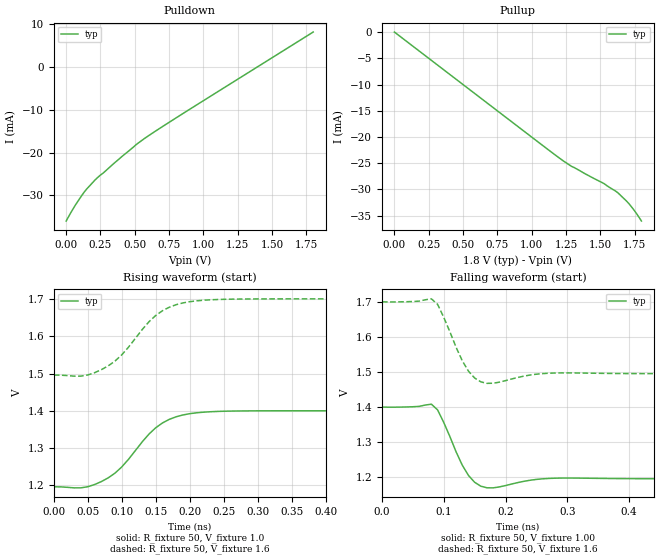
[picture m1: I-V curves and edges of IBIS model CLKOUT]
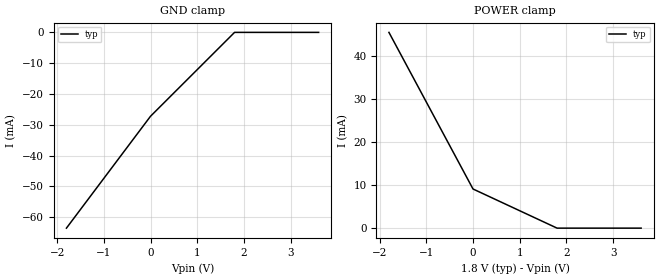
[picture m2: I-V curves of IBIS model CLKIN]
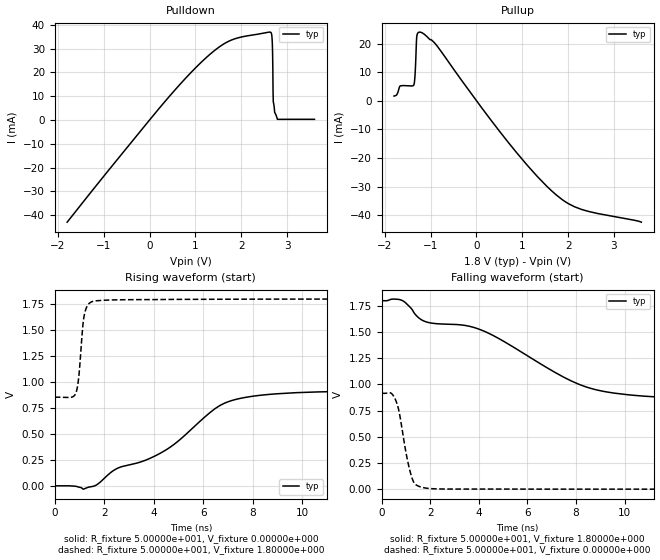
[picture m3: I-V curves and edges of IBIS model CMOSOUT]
|This Model applies to CDCL1810 and CDCL1810A Clock Buffers
[IBIS Ver] 4.0
[Comment char] |_char
[File Name] cdcl1810a.ibs
[File Rev] 2.0
[Source] Texas Instruments, Inc. Created from TISpice model
[Date] March 01, 2006
[Disclaimer]
|*   Property of Texas Instruments Incorporated.  Unauthorized  *
|*   reproduction and/or distribution is strictly prohibited.   *
|*   This product is protected under copyright law.   *
|*   (C) Copyright 2006, Texas Instruments Inc.,   *
|*   All Rights Reserved   *
|*   UNLESS THERE IS A SIGNED, WRITTEN AGREEMENT TO THE   *
|*   CONTRARY, TEXAS INSTRUMENTS ("TI") IS PROVIDING THE SPICE  *
|*   MODELS "AS IS" AND WITHOUT ANY WARRANTY, EXPRESSED OR   *
|*   IMPLIED.  TI assumes no liability for:   *
|*   1) the accuracy of the IBIS models provided to your   *
|*   company;   *
|*   2) the proper functioning of these IBIS models in your   *
|*   design or for any resulting applications; or   *
|*   3) infringement of patents, copyrights or intellectual   *
|*   property rights resulting from your use of these   *
|*   IBIS models.   *
|*   TI provides IBIS Models as a service to our customers.   *
|*   You and your company shall not distribute, sell or give   *
|*   these models to anyone else without prior written   *
|*   permission from TI.   *
|*   TI reserves the right to make changes to our products or   *
|*   to discontinue any semiconductor product or service   *
|*   without notice, and advises our customers to obtain the   *
|*   latest version of relevant information to verify, before   *
|*   placing orders, that the information being relied on is   *
|*   current.   *
|*   Please be aware that your receipt and use of the IBIS   *
|*   information provided shall serve as acceptance of these   *
|*   terms and conditions.  If you do not accept these terms,   *
|*   you should return or destroy the IBIS models and any   *
|*   other accompanying information immediately.   *
[Component] CDCL1810A
[Manufacturer] Texas Instruments, Inc.
[Package]
| variable   typ   min  max
R_pkg   0.175ohm   NA   NA
L_pkg   2.081nH   NA   NA
C_pkg   0.045pF   NA   NA
[Pin]   signal_name   model_name   R_pin   L_pin   C_pin
2   AVDD   POWER   NA   NA   NA
3   CLKP   CLKIN   NA   NA   NA
4   CLKN   CLKIN   NA   NA   NA
5   AVDD   POWER   NA   NA   NA
6   YP0   CLKOUT   NA   NA   NA
7   YN0   CLKOUT   NA   NA   NA
8   VDD   POWER   NA   NA   NA
9   YP1   CLKOUT   NA   NA   NA
10   YN1   CLKOUT   NA   NA   NA
11   VDD   POWER   NA   NA   NA
12   GND   GND   NA   NA   NA
13   STATUS   CMOSOUT   NA   NA   NA
14   VDD   POWER   NA   NA   NA
15   YP2   CLKOUT   NA   NA   NA
16   YN2   CLKOUT   NA   NA   NA
17   VDD   POWER   NA   NA   NA
18   YP3   CLKOUT   NA   NA   NA
19   YN3   CLKOUT   NA   NA   NA
20   VDD   POWER   NA   NA   NA
21   YP4   CLKOUT   NA   NA   NA
22   YN4   CLKOUT   NA   NA   NA
23   VDD   POWER   NA   NA   NA
24   SCL   CMOSIN   NA   NA   NA
25   SDA   CMOSIO   NA   NA   NA
26   VDD   POWER   NA   NA   NA
27   YP5   CLKOUT   NA   NA   NA
28   YN5   CLKOUT   NA   NA   NA
29   VDD   POWER   NA   NA   NA
30   YP6   CLKOUT   NA   NA   NA
31   YN6   CLKOUT   NA   NA   NA
32   VDD   POWER   NA   NA   NA
33   YP7   CLKOUT   NA   NA   NA
34   YN7   CLKOUT   NA   NA   NA
35   VDD   POWER   NA   NA   NA
36   ADD0   CMOSIN   NA   NA   NA
37   ADD1   CMOSIN   NA   NA   NA
38   VDD   POWER   NA   NA   NA
39   YN8   CLKOUT   NA   NA   NA
40   YP8   CLKOUT   NA   NA   NA
41   VDD   POWER   NA   NA   NA
42   YN9   CLKOUT   NA   NA   NA
43   YP9   CLKOUT   NA   NA   NA
44   AVDD   POWER   NA   NA   NA
45   YN10   CLKOUT   NA   NA   NA
46   YP10   CLKOUT   NA   NA   NA
47   AVDD   POWER   NA   NA   NA
[Diff Pin]   inv_pin  vdiff   tdelay_typ  tdelay_min  tdelay_max
3   4   100mV   NA   NA   NA
6   7   100mV   NA   NA   NA
9   10   100mV   NA   NA   NA
15   16   100mV   NA   NA   NA
18   19   100mV   NA   NA   NA
21   22   100mV   NA   NA   NA
27   28   100mV   NA   NA   NA
30   31   100mV   NA   NA   NA
33   34   100mV   NA   NA   NA
40   39   100mV   NA   NA   NA
43   42   100mV   NA   NA   NA
46   45   100mV   NA   NA   NA
[Series Pin Mapping]   pin_2   model_name  function_table_group
3   4   RTERM
6   7   CDIFFOUT
9   10   CDIFFOUT
15   16   CDIFFOUT
18   19   CDIFFOUT
21   22   CDIFFOUT
27   28   CDIFFOUT
30   31   CDIFFOUT
33   34   CDIFFOUT
40   39   CDIFFOUT
43   42   CDIFFOUT
46   45   CDIFFOUT
|   Model CDIFFOUT
[Model] CDIFFOUT
Model_type Series
Polarity Non-Inverting
Enable  Active-High
| variable   typ   min   max
C_comp   0.0000pF   NA   NA
[Voltage Range]   1.8000V   NA   NA
[POWER Clamp Reference]   1.8000V   NA   NA
[GND Clamp Reference]   0.0000V   NA   NA
|   C(typ)   C(min)   C(max)
[C Series]   0.08pF   NA   NA
|   Model RTERM
[Model] RTERM
Model_type Series
Polarity Non-Inverting
Enable  Active-High
| variable   typ   min   max
C_comp   0.0000pF  NA   NA
[Voltage Range]   1.8000V   NA   NA
[POWER Clamp Reference]   1.8000V   NA   NA
[GND Clamp Reference]   0.0000V   NA   NA
|   R(typ)   R(min)   R(max)
[R Series]   100ohm   NA   NA
| Models and submodels in the file (7): CLKOUT (Output), CDIFFOUT (Series), CLKIN (Input), RTERM (Series), CMOSOUT (Output), CMOSIO (I/O), CMOSIN (Input)
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|   Model CLKOUT
[Model] CLKOUT
Model_type Output
Polarity Non-Inverting
Vmeas  = 1.40000e+000
Cref   = 0.00000e+000
Rref   = 5.00000e+001
Vref   = 1.20000e+000
|   typ   min   max
C_comp   2.00000e-013   2.00000e-013   2.00000e-013
[Temperature Range]   2.70000e+001   8.50000e+001   -4.00000e+001
|   typ   min   max
[Voltage Range]   1.80000e+000   1.70000e+000   1.90000e+000
[Pullup Reference]   1.80000e+000   1.80000e+000   1.80000e+000
[Pulldown Reference]   0.00000e+000   0.00000e+000   0.00000e+000
[POWER Clamp Reference]   1.80000e+000   1.80000e+000   1.80000e+000
[GND Clamp Reference]   0.00000e+000   0.00000e+000   0.00000e+000
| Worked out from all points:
|   slope of the pulldown table from 0 to 0.27 V, typ, clamps not added: 24 ohm
|   slope of the pullup table from 0 to 0.27 V, typ, clamps not added: 50 ohm
|   falling waveform, R_fixture 50, V_fixture 1.00: 20-80 % time 30.2ps typ, NA min, NA max; typ from 1.4 V to 1.2 V
|   falling waveform, R_fixture 50, V_fixture 1.6: 20-80 % time 29.7ps typ, NA min, NA max; typ from 1.7 V to 1.5 V
|   rising waveform, R_fixture 50, V_fixture 1.0: 20-80 % time 61.2ps typ, NA min, NA max; typ from 1.2 V to 1.4 V
|   rising waveform, R_fixture 50, V_fixture 1.6: 20-80 % time 60.8ps typ, NA min, NA max; typ from 1.5 V to 1.7 V
[Pullup]
| Voltage   I(typ)   I(min)   I(max)
0V        173.6nA    NA         NA
1.23V     -24.54mA   NA         NA
1.29V     -25.58mA   NA         NA
1.53V     -28.93mA   NA         NA
1.63V     -30.67mA   NA         NA
1.71V     -32.73mA   NA         NA
1.75V     -34.06mA   NA         NA
1.8V      -36.02mA   NA         NA
[Pulldown]
| Voltage   I(typ)   I(min)   I(max)
0V        -36.02mA   NA         NA
70mV      -32.14mA   NA         NA
150mV     -28.51mA   NA         NA
230mV     -25.81mA   NA         NA
510mV     -18.14mA   NA         NA
610mV     -15.85mA   NA         NA
790mV     -12.12mA   NA         NA
1.8V      8.186mA    NA         NA
[Ramp]
R_load = 5.000e+001
|   typ   min   max
dV/dt_r  0.11E+00/6.01E-11   NA   NA
dV/dt_f  0.11E+00/4.01E-11   NA   NA
[Falling Waveform]
R_fixture=50
C_fixture=0p
V_fixture=1.00
V_fixture_min=1.00
V_fixture_max=1.00
|Time   Typ   Min   Max
|SECONDS   VOLTS   VOLTS   VOLTS
0s        1.4V       NA         NA
80ps      1.408V     NA         NA
90ps      1.392V     NA         NA
130ps     1.234V     NA         NA
140ps     1.205V     NA         NA
160ps     1.175V     NA         NA
180ps     1.17V      NA         NA
240ps     1.192V     NA         NA
300ps     1.198V     NA         NA
35ns      1.196V     NA         NA
[Falling Waveform]
R_fixture=50
C_fixture=0p
V_fixture=1.6
V_fixture_min=1.6
V_fixture_max=1.6
|Time   Typ   Min   Max
|SECONDS   VOLTS   VOLTS   VOLTS
0s        1.7V       NA         NA
80ps      1.708V     NA         NA
90ps      1.693V     NA         NA
130ps     1.532V     NA         NA
140ps     1.502V     NA         NA
150ps     1.483V     NA         NA
170ps     1.468V     NA         NA
240ps     1.491V     NA         NA
290ps     1.497V     NA         NA
35ns      1.496V     NA         NA
[Rising Waveform]
R_fixture=50
C_fixture=0p
V_fixture=1.0
V_fixture_min=1.0
V_fixture_max=1.0
|Time   Typ   Min   Max
|SECONDS   VOLTS   VOLTS   VOLTS
0s        1.196V     NA         NA
50ps      1.197V     NA         NA
80ps      1.22V      NA         NA
100ps     1.25V      NA         NA
130ps     1.317V     NA         NA
150ps     1.355V     NA         NA
180ps     1.384V     NA         NA
220ps     1.396V     NA         NA
300ps     1.4V       NA         NA
35ns      1.4V       NA         NA
[Rising Waveform]
R_fixture=50
C_fixture=0p
V_fixture=1.6
V_fixture_min=1.6
V_fixture_max=1.6
|Time   Typ   Min   Max
|SECONDS   VOLTS   VOLTS   VOLTS
0s        1.496V     NA         NA
40ps      1.493V     NA         NA
60ps      1.502V     NA         NA
80ps      1.52V      NA         NA
100ps     1.55V      NA         NA
140ps     1.639V     NA         NA
170ps     1.678V     NA         NA
210ps     1.695V     NA         NA
300ps     1.7V       NA         NA
35ns      1.7V       NA         NA
[Model]   CLKIN
Model_type   Input
Vinl   = 6.00000e-001
Vinh   = 1.20000e+000
|   typ   min   max
C_comp   1.00000e-012   1.00000e-012   1.00000e-012
[Temperature Range]   2.70000e+001   NA   NA
|   |   typ   min   max
[Voltage Range]   1.80000e+000   NA   NA
[Pullup Reference]   1.80000e+000   NA   NA
[Pulldown Reference]   0.00000e+000   NA   NA
[POWER Clamp Reference]   1.80000e+000   NA   NA
[GND Clamp Reference]   0.00000e+000   NA   NA
[GND Clamp]
| Voltage   I(typ)   I(min)   I(max)
-1.8V     -63.55mA   NA         NA
1.52fV    -27.24mA   NA         NA
1.8V      0A         NA         NA
3.6V      0A         NA         NA
[POWER Clamp]
| Voltage   I(typ)   I(min)   I(max)
-1.8V     45.39mA    NA         NA
1.52fV    9.077mA    NA         NA
1.8V      0A         NA         NA
3.6V      0A         NA         NA
|   Model CMOSOUT
[Model]   CMOSOUT
Model_type   Output
Vmeas  = 9.00000e-001
Cref   = 0.00000e+000
Rref   = 2.50000e+001
Vref   = 9.00000e-001
|   typ   min   max
C_comp   9.00000e-013   9.00000e-013   9.00000e-013
[Temperature Range]   2.70000e+001   NA   NA
|   |   typ   min   max
[Voltage Range]   1.80000e+000   NA   NA
[Pullup Reference]   1.80000e+000   NA   NA
[Pulldown Reference]   0.00000e+000   NA   NA
[POWER Clamp Reference]   1.80000e+000   NA   NA
[GND Clamp Reference]   0.00000e+000   NA   NA
[Ramp]
R_load = 5.000e+001
|   typ   min   max
dV/dt_r 5.494e-001/3.727e-009   NA   NA
dV/dt_f 5.677e-001/6.028e-009   NA   NA
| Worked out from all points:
|   slope of the pulldown table from 0 to 0.27 V, typ, clamps not added: 43.1 ohm
|   slope of the pullup table from 0 to 0.27 V, typ, clamps not added: 46.4 ohm
|   rising waveform, R_fixture 5.00000e+001, V_fixture 0.00000e+000: 20-80 % time 3.73ns typ, NA min, NA max; typ from 0 V to 0.916 V
|   rising waveform, R_fixture 5.00000e+001, V_fixture 1.80000e+000: 20-80 % time 201ps typ, NA min, NA max; typ from 0.854 V to 1.8 V
|   falling waveform, R_fixture 5.00000e+001, V_fixture 1.80000e+000: 20-80 % time 6.03ns typ, NA min, NA max; typ from 1.8 V to 0.854 V
|   falling waveform, R_fixture 5.00000e+001, V_fixture 0.00000e+000: 20-80 % time 431ps typ, NA min, NA max; typ from 0.916 V to 0 V
[Pullup]
| Voltage   I(typ)   I(min)   I(max)
-1.8V     1.64mA     NA         NA
-1.665V   5.16mA     NA         NA
-1.365V   5.627mA    NA         NA
-1.34V    9.3mA      NA         NA
-1.31V    20.92mA    NA         NA
-1.3V     22.86mA    NA         NA
-1.19V    23.8mA     NA         NA
-870mV    19.39mA    NA         NA
865mV     -17.94mA   NA         NA
1.725V    -32.72mA   NA         NA
2.295V    -38.03mA   NA         NA
3.6V      -42.49mA   NA         NA
[Pulldown]
| Voltage   I(typ)   I(min)   I(max)
-1.8V     -42.96mA   NA         NA
655mV     14.78mA    NA         NA
1.78V     33.53mA    NA         NA
2.65V     36.71mA    NA         NA
2.68V     31.72mA    NA         NA
2.685V    28.09mA    NA         NA
2.69V     21.96mA    NA         NA
2.695V    11.81mA    NA         NA
2.7V      7.614mA    NA         NA
2.73V     3.249mA    NA         NA
2.79V     265.3uA    NA         NA
3.6V      271.9uA    NA         NA
[Rising Waveform]
R_fixture   = 5.00000e+001
V_fixture   = 0.00000e+000
C_fixture   = 0.00000e+000
| Time   V(typ)   V(min)   V(max)
0s        760.5nV    NA         NA
1.15ns    -32.43mV   NA         NA
1.65ns    3.737mV    NA         NA
2.5ns     164.9mV    NA         NA
3.625ns   242.7mV    NA         NA
4.475ns   342.8mV    NA         NA
6.45ns    738.5mV    NA         NA
7.325ns   833mV      NA         NA
9.75ns    897.5mV    NA         NA
14.98ns   915.7mV    NA         NA
[Rising Waveform]
R_fixture   = 5.00000e+001
V_fixture   = 1.80000e+000
C_fixture   = 0.00000e+000
| Time   V(typ)   V(min)   V(max)
0s        853.9mV    NA         NA
675ps     853.7mV    NA         NA
850ps     892.1mV    NA         NA
925ps     966.4mV    NA         NA
975ps     1.061V     NA         NA
1.125ns   1.52V      NA         NA
1.2ns     1.655V     NA         NA
1.325ns   1.738V     NA         NA
1.55ns    1.778V     NA         NA
14.98ns   1.8V       NA         NA
[Falling Waveform]
R_fixture   = 5.00000e+001
V_fixture   = 1.80000e+000
C_fixture   = 0.00000e+000
| Time   V(typ)   V(min)   V(max)
0s        1.8V       NA         NA
850ps     1.801V     NA         NA
1.5ns     1.641V     NA         NA
1.85ns    1.596V     NA         NA
3.4ns     1.564V     NA         NA
4.175ns   1.512V     NA         NA
7.45ns    1.075V     NA         NA
8.675ns   958mV      NA         NA
10.87ns   886.9mV    NA         NA
14.98ns   853.9mV    NA         NA
[Falling Waveform]
R_fixture   = 5.00000e+001
V_fixture   = 0.00000e+000
C_fixture   = 0.00000e+000
| Time   V(typ)   V(min)   V(max)
0s        915.7mV    NA         NA
375ps     918.1mV    NA         NA
575ps     851mV      NA         NA
725ps     731.6mV    NA         NA
1.025ns   320.7mV    NA         NA
1.225ns   124.8mV    NA         NA
1.375ns   48.56mV    NA         NA
1.65ns    18.16mV    NA         NA
2.7ns     1.24mV     NA         NA
14.98ns   760.5nV    NA         NA
